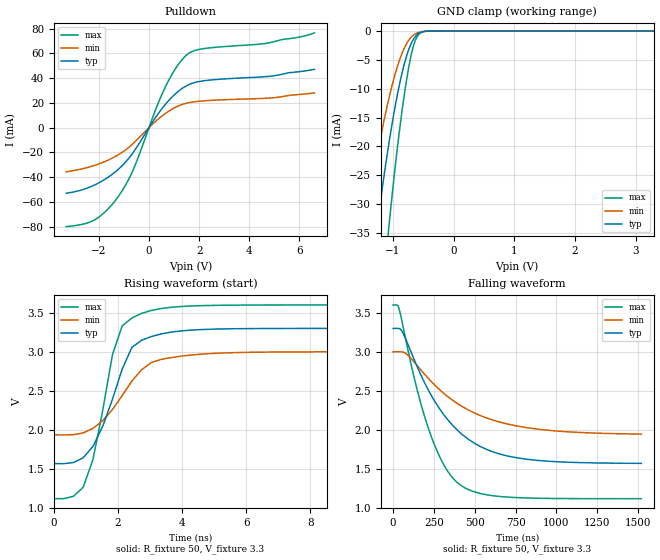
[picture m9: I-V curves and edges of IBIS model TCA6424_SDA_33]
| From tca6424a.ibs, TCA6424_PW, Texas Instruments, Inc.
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[Model]   TCA6424_SDA_33
Model_type  I/O_open_drain
Vinl=0.9
Vinh=2.52
Enable   Active-Low
Vref =   0
Rref =   500
Cref =   50p
Vmeas =   1.65
| variable   typ   min   max
C_comp   3.09pF   2.16pF   3.48pF
| C_pulldown   1.93pF   0.71pF   2.60pF
| C_tri-state   3.09pF   2.16pF   3.48pF
[Temperature Range]   40   100   -40
| Ambient temperature   25   85   -40
[Voltage range]   3.3   3   3.6
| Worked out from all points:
|   slope of the pulldown table from 0 to 0.495 V, typ, clamps not added: 33.5 ohm
|   GND clamp passes 1 mA (typ) near -0.63 V on its own axis
|   rising waveform, R_fixture 50, V_fixture 3.3: 20-80 % time 952ps typ, 1.2ns min, 728ps max; typ from 1.57 V to 3.3 V
|   falling waveform, R_fixture 50, V_fixture 3.3: 20-80 % time 319ns typ, 406ns min, 212ns max; typ from 3.3 V to 1.57 V
[GND Clamp]
| TCA6424_SDA_33
|   Voltage   I(typ)   I(min)   I(max)
-3.3V     -264.2mA   -197.1mA   -365.9mA
-1.46V    -51.4mA    -34.15mA   -81.8mA
-1.26V    -34.01mA   -21.73mA   -56.19mA
-1.075V   -20.18mA   -12.16mA   -35mA
-1.06V    -19.18mA   -11.48mA   -33.41mA
-940mV    -11.86mA   -6.678mA   -21.61mA
-815mV    -5.875mA   -3.052mA   -11.35mA
-710mV    -2.471mA   -1.225mA   -4.762mA
-615mV    -792.7uA   -414.6uA   -1.278mA
-540mV    -234.4uA   -145.4uA   -292.5uA
-410mV    -16.25uA   -13.51uA   -13.24uA
3.3V      403.3pA    1.225nA    137.8pA
[Pulldown]
| TCA6424_SDA_33
|   Voltage   I(typ)   I(min)   I(max)
-3.3V     -52.99mA   -35.6mA    -79.91mA
-2.15V    -46.11mA   -30.34mA   -74.26mA
-1.685V   -40.79mA   -26.72mA   -66.72mA
-1.22V    -33.58mA   -21.85mA   -55.5mA
-630mV    -20.06mA   -12.81mA   -34.11mA
255mV     8.017mA    4.951mA    14.05mA
670mV     19.21mA    11.72mA    33.54mA
1.115V    28.43mA    17.02mA    49.47mA
1.535V    34.24mA    19.97mA    59.3mA
2.105V    37.65mA    21.54mA    63.61mA
4.625V    41.18mA    23.71mA    67.98mA
6.6V      47.17mA    28.14mA    76.63mA
[Ramp]
| TCA6424_SDA_33
| variable   typ   min   max
dV/dt_r   1.04/9.11E-10   0.64/1.19E-09   1.49/6.85E-10
dV/dt_f   1.04/3.19E-07   0.63/4.06E-07   1.49/2.12E-07
R_load = 50
[Rising Waveform]
| TCA6424_SDA_33
R_fixture =   50
C_fixture =   0
L_fixture =   0
V_fixture =   3.3
V_fixture_min = 3
V_fixture_max = 3.6
|   Time   V(typ)   V(min)   V(max)
0s        1.57V      1.939V     1.12V
917ps     1.642V     1.961V     1.264V
1.221ns   1.788V     2.018V     1.619V
1.525ns   2.044V     2.116V     2.247V
1.829ns   2.39V      2.259V     2.96V
2.133ns   2.777V     2.438V     3.333V
2.437ns   3.056V     2.626V     3.433V
3.045ns   3.195V     2.862V     3.53V
6.085ns   3.296V     2.993V     3.598V
1.52us    3.3V       3V         3.6V
[Falling Waveform]
| TCA6424_SDA_33
R_fixture =   50
C_fixture =   0
L_fixture =   0
V_fixture =   3.3
V_fixture_min = 3
V_fixture_max = 3.6
|   Time   V(typ)   V(min)   V(max)
0s        3.3V       3V         3.6V
36.18ns   3.299V     3.001V     3.555V
64.45ns   3.224V     2.995V     3.29V
144.7ns   2.824V     2.832V     2.535V
235.3ns   2.437V     2.617V     1.907V
313.1ns   2.188V     2.464V     1.542V
404ns     1.977V     2.325V     1.307V
557.2ns   1.765V     2.166V     1.176V
752.7ns   1.645V     2.053V     1.134V
1.52us    1.573V     1.947V     1.12V
